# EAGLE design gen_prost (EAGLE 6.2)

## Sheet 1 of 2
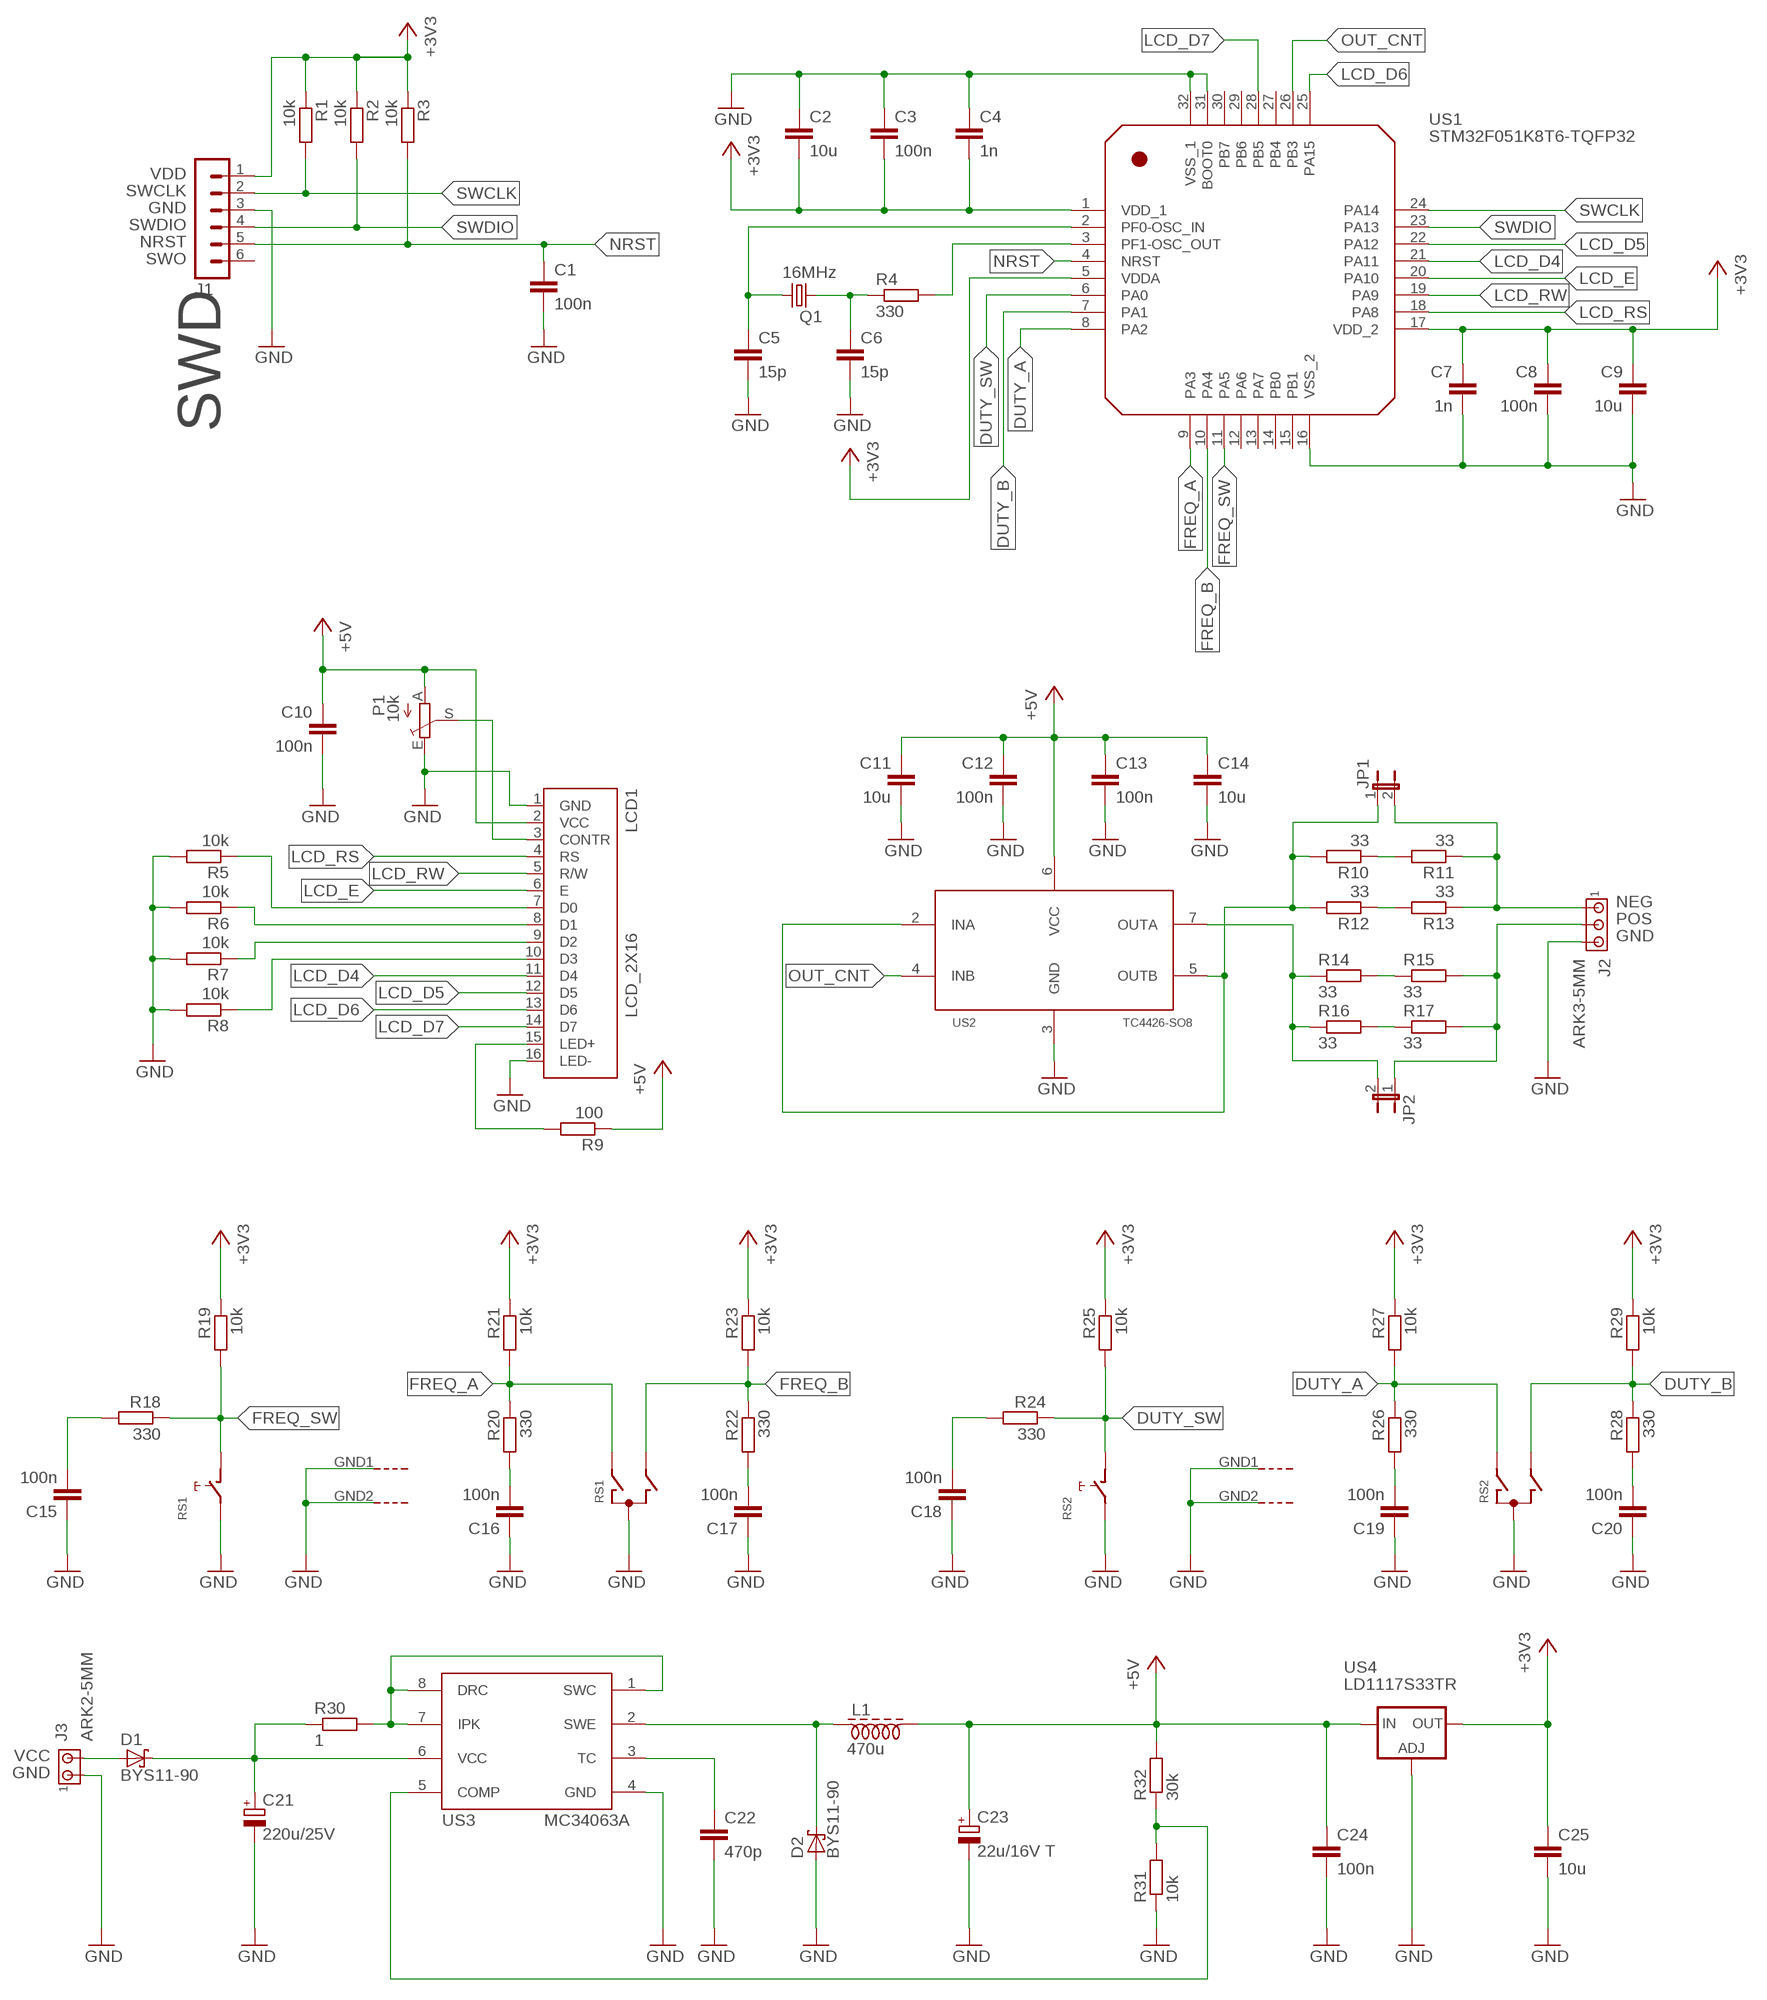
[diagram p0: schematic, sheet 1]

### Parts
C1  100n  C-EUC0805K  [C0805K]
C2  10u  C-EUC0805K  [C0805K]
C3  100n  C-EUC0805K  [C0805K]
C4  1n  C-EUC0805K  [C0805K]
C5  15p  C-EUC0805K  [C0805K]
C6  15p  C-EUC0805K  [C0805K]
C7  1n  C-EUC0805K  [C0805K]
C8  100n  C-EUC0805K  [C0805K]
C9  10u  C-EUC0805K  [C0805K]
C10  100n  C-EUC0805K  [C0805K]
C11  10u  C-EUC0805K  [C0805K]
C12  100n  C-EUC0805K  [C0805K]
C13  100n  C-EUC0805K  [C0805K]
C14  10u  C-EUC0805K  [C0805K]
C15  100n  C-EUC0805K  [C0805K]
C16  100n  C-EUC0805K  [C0805K]
C17  100n  C-EUC0805K  [C0805K]
C18  100n  C-EUC0805K  [C0805K]
C19  100n  C-EUC0805K  [C0805K]
C20  100n  C-EUC0805K  [C0805K]
C21  220u/25V  CPOL-EUTT5D7L  [TT5D7L]
C22  470p  C-EUC0805  [C0805]
C23  22u/16V T  CPOL-EUSMCC  [SMC_C]
C24  100n  C-EUC0805K  [C0805K]
C25  10u  C-EUC0805K  [C0805K]
D1  BYS11-90  SCHOTTKY-DIODESMD  [SMB]
D2  BYS11-90  SCHOTTKY-DIODESMD  [SMB]
J1  MA06-1  [MA06-1]
J2  ARK3-5MM  [3PIN-5MM]
J3  ARK2-5MM  [2PIN-5MM]
JP1  JP1E  [JP1]
JP2  JP1E  [JP1]
L1  470u  DLAWIK-PION  [L_PION]
LCD1  LCD_2X16  LCD_2X16-NAD-ELEMENTAMI  [LCD_HD44780_2X16_NAD-ELEMENTAMI]
P1  10k  TRIM_EU-CA6V  [CA6V]
Q1  16MHz  CRYSTALSM49  [SM49]
R1  10k  R-EU_M0805  [M0805]
R2  10k  R-EU_M0805  [M0805]
R3  10k  R-EU_M0805  [M0805]
R4  330  R-EU_M0805  [M0805]
R5  10k  R-EU_M0805  [M0805]
R6  10k  R-EU_M0805  [M0805]
R7  10k  R-EU_M0805  [M0805]
R8  10k  R-EU_M0805  [M0805]
R9  100  R-EU_M0805  [M0805]
R10  33  R-EU_M0805  [M0805]
R11  33  R-EU_M0805  [M0805]
R12  33  R-EU_M0805  [M0805]
R13  33  R-EU_M0805  [M0805]
R14  33  R-EU_M0805  [M0805]
R15  33  R-EU_M0805  [M0805]
R16  33  R-EU_M0805  [M0805]
R17  33  R-EU_M0805  [M0805]
R18  330  R-EU_M0805  [M0805]
R19  10k  R-EU_M0805  [M0805]
R20  330  R-EU_M0805  [M0805]
R21  10k  R-EU_M0805  [M0805]
R22  330  R-EU_M0805  [M0805]
R23  10k  R-EU_M0805  [M0805]
R24  330  R-EU_M0805  [M0805]
R25  10k  R-EU_M0805  [M0805]
R26  330  R-EU_M0805  [M0805]
R27  10k  R-EU_M0805  [M0805]
R28  330  R-EU_M0805  [M0805]
R29  10k  R-EU_M0805  [M0805]
R30  1  R-EU_M0805  [M0805]
R31  10k  R-EU_M0805  [M0805]
R32  30k  R-EU_M0805  [M0805]
RS1  EC12E_SW  [ALPS_EC12E_SW]
RS2  EC12E_SW  [ALPS_EC12E_SW]
US1  STM32F051K8T6-TQFP32  STM32F051-TQFP32  [TQFP32]
US2  TC4426-SO8  [SO08]
US3  MC34063A  MC34063-SO8  [SO08@1]
US4  LD1117S33TR  LD117AS33TR  [SOT223]

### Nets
+3V3: C2.2 C3.2 C4.2 C7.1 C8.1 C9.1 C25.1 J1.1 R1.1 R2.1 R3.1 R19.1 R21.1 R23.1 R25.1 R27.1 R29.1 US1.1(VDD_1) US1.5(VDDA) US1.17(VDD_2) US4.4(OUT)
+5V: C10.1 C11.1 C12.1 C13.1 C14.1 C23.+ C24.1 L1.P$2 LCD1.2(VCC) P1.A R9.1 R32.2 US2.6(VCC) US4.3(IN)
DUTY_A: R26.1 R27.2 RS2.A US1.8(PA2)
DUTY_B: R28.1 R29.2 RS2.B US1.7(PA1)
DUTY_SW: R24.1 R25.2 RS2.D US1.6(PA0)
FREQ_A: R20.1 R21.2 RS1.A US1.9(PA3)
FREQ_B: R22.1 R23.2 RS1.B US1.10(PA4)
FREQ_SW: R18.1 R19.2 RS1.D US1.11(PA5)
GND: C1.2 C2.1 C3.1 C4.1 C5.2 C6.2 C7.2 C8.2 C9.2 C10.2 C11.2 C12.2 C13.2 C14.2 C15.1 C16.1 C17.1 C18.1 C19.1 C20.1 C21.- C22.2 C23.- C24.2 C25.2 D2.A J1.3 J2.P$3 J3.P$1 LCD1.1(GND) LCD1.16(LED-) P1.E R5.2 R6.2 R7.2 R8.2 R31.1 RS1.C RS1.E RS1.GND1(G) RS1.GND2(G) RS2.C RS2.E RS2.GND1(G) RS2.GND2(G) US1.16(VSS_2) US1.31(BOOT0) US1.32(VSS_1) US2.3(GND) US3.4(GND) US4.1(ADJ)
LCD_D4: LCD1.11(D4) US1.21(PA11)
LCD_D5: LCD1.12(D5) US1.22(PA12)
LCD_D6: LCD1.13(D6) US1.25(PA15)
LCD_D7: LCD1.14(D7) US1.28(PB5)
LCD_E: LCD1.6(E) US1.20(PA10)
LCD_RS: LCD1.4(RS) US1.18(PA8)
LCD_RW: LCD1.5(R/W) US1.19(PA9)
N$1: R31.2 R32.1 US3.5(COMP)
N$2: C18.2 R24.2
N$3: C19.2 R26.2
N$4: C20.2 R28.2
N$5: JP2.2 R14.1 R16.1 US2.7(OUTA)
N$6: R10.1 R11.2
N$7: R12.1 R13.2
N$8: J2.P$1 JP1.2 R11.1 R13.1
N$9: JP1.1 R10.2 R12.2 US2.2(INA) US2.5(OUTB)
N$10: C15.2 R18.2
N$11: J2.P$2 JP2.1 R15.2 R17.2
N$12: C16.2 R20.2
N$13: C17.2 R22.2
N$14: LCD1.9(D2) R7.1
N$16: R16.2 R17.1
N$17: R14.2 R15.1
N$23: C5.1 Q1.1 US1.2(PF0-OSC_IN)
N$24: LCD1.15(LED+) R9.2
N$25: LCD1.3(CONTR) P1.S
N$26: LCD1.8(D1) R6.1
N$27: LCD1.7(D0) R5.1
N$28: LCD1.10(D3) R8.1
N$31: D1.A J3.P$2
N$32: C21.+ D1.C R30.1 US3.6(VCC)
N$37: R30.2 US3.1(SWC) US3.7(IPK) US3.8(DRC)
N$38: C22.1 US3.3(TC)
N$39: D2.C L1.P$1 US3.2(SWE)
N$71: R4.2 US1.3(PF1-OSC_OUT)
N$72: C6.1 Q1.2 R4.1
NRST: C1.1 J1.5 R3.2 US1.4(NRST)
OUT_CNT: US1.26(PB3) US2.4(INB)
SWCLK: J1.2 R1.2 US1.24(PA14)
SWDIO: J1.4 R2.2 US1.23(PA13)
Unconnected: J1.6 US1.12(PA6) US1.13(PA7) US1.14(PB0) US1.15(PB1) US1.27(PB4) US1.29(PB6) US1.30(PB7)

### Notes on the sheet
- VDD
- SWCLK
- GND
- SWDIO
- NRST
- SWO
- SWD
- NEG
- POS
- GND
- VCC
- GND

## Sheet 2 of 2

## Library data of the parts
C1-C20 C22 C24 C25 = rcl:C-EU: CAPACITOR, European symbol
C21 C23 = rcl:CPOL-EU: POLARIZED CAPACITOR, European symbol
D1 D2 = diode:SCHOTTKY-DIODE: Schottky Diode
J1 = con-lstb:MA06-1: PIN HEADER; OC_FARNELL: unknown; OC_NEWARK: unknown
J2 = zlacza_futrzak:ARK3: ARK 3 Raster 5mm i 3,5mm
J3 = zlacza_futrzak:ARK2: ARK 2
JP1 JP2 = jumper:JP1E: JUMPER
L1 = inne_futrzak:DLAWIK
LCD1 = inne_futrzak:LCD_2X16
P1 = pot:TRIM_EU-: POTENTIOMETER
Q1 = crystal:CRYSTAL: CRYSTAL; OC_FARNELL: unknown; OC_NEWARK: unknown
R1-R32 = rcl:R-EU_: RESISTOR, European symbol
RS1 RS2 = switch-alps:EC12E_SW: ALPS rotary Encoder EC12E series with switch; MPN: EC12E2424407; OC_FARNELL: 1520813; OC_NEWARK: 74M1068
US1 = scalaki_futrzak:STM32F051-TQFP32
US2 = scalaki_futrzak:TC4426
US3 = scalaki_futrzak:MC34063
US4 = v-reg:LD117A?*: Low drop fixed and adjustable positive voltage regulators 1 A Source: http://www.st.com/stonline/products/literature/ds/7194/ld1117axx.pdf

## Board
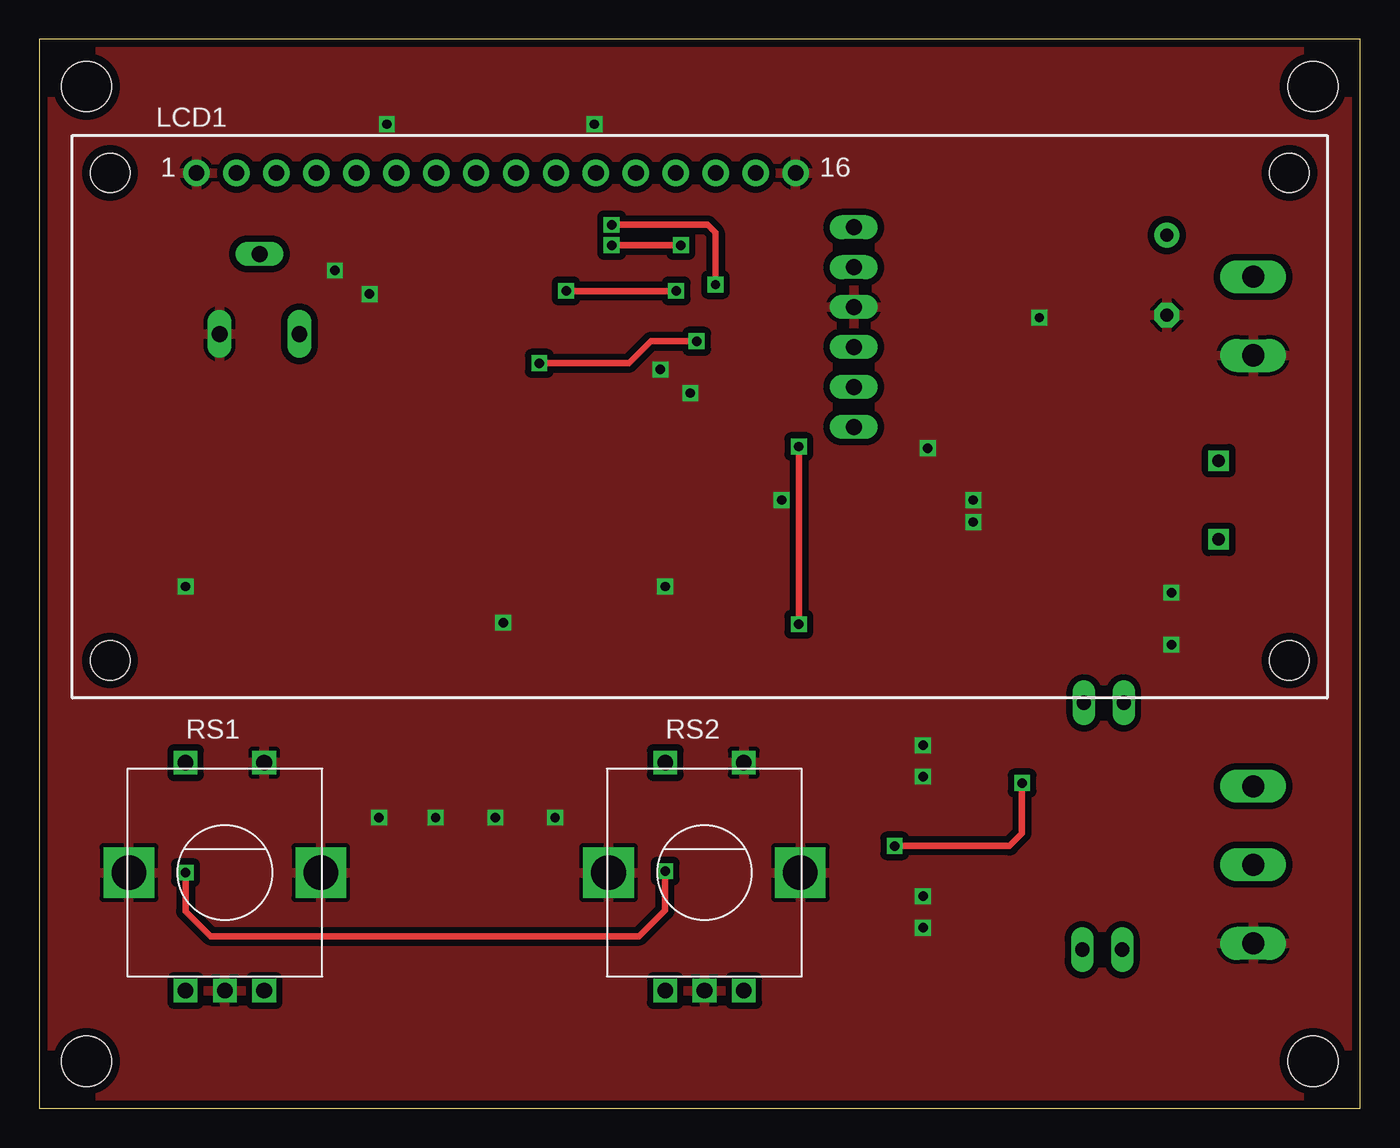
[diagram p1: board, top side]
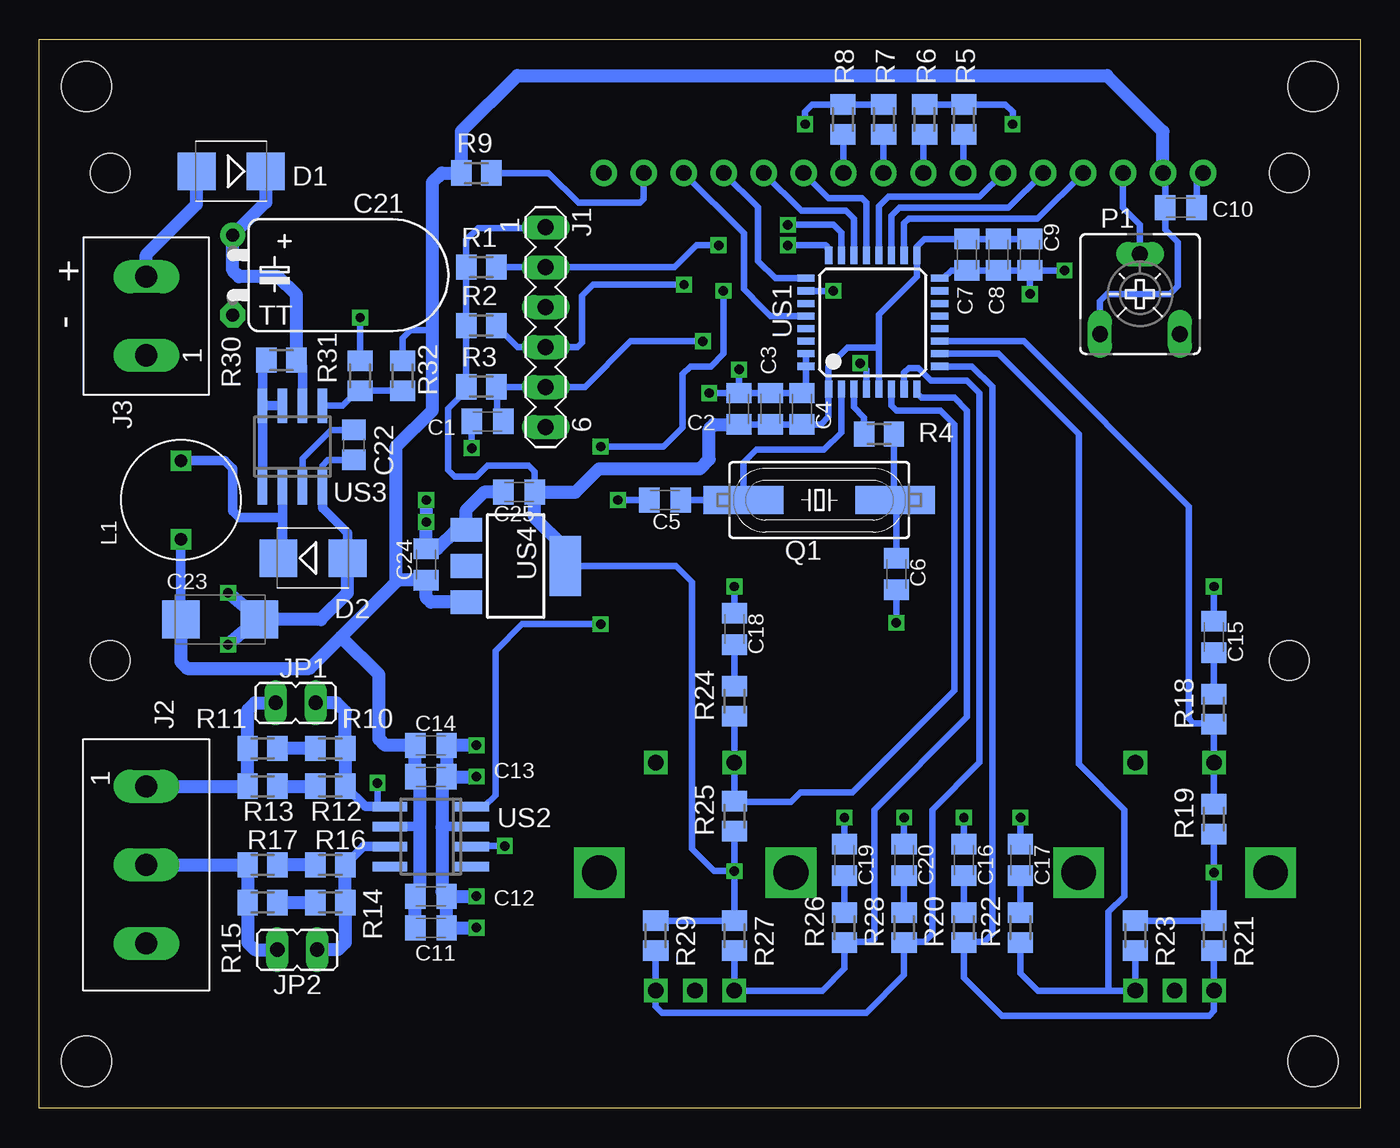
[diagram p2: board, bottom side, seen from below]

Size 84 x 68 mm. Coordinates in mm from the lower left corner, seen from the top.
Outline: 0,0 84,0 84,68 0,68 0,0
Copper layers (1*16): Top 0.035mm / dielectric 1.5mm / Bottom 0.035mm
Design rules: minimum track width 10mil, minimum drill 23mil, track to track 8mil, track to pad 8mil, pad to pad 8mil, via to via 8mil, smd to smd 8mil, copper to edge 20mil, drill to drill 8mil, minimum pad ring 10mil, minimum via ring 8mil, stop-mask expansion 4mil, vias tented up to drill 0mil, thermal gap 10mil
Holes 3.2 mm at 3,3 81,3 3,65 81,65

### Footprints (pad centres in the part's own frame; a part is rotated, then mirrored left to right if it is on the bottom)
C0805K = smd 1.3 x 1.6: 1 -1,0; 2 1,0
TT5D7L = drill 0.813 pad 1.6: + -2.54,0 | drill 0.813 pad 1.6 octagon: - 2.54,0
C0805 = smd 1.3 x 1.5: 1 -0.95,0; 2 0.95,0
SMC_C = smd 2.4 x 2.4: + -2.5,0; - 2.5,0
SMB = smd 2.4 x 2.4: A 2.2,0; C -2.2,0
MA06-1 = drill 1.016 long: 1 -6.35,0; 2 -3.81,0; 3 -1.27,0; 4 1.27,0; 5 3.81,0; 6 6.35,0
3PIN-5MM = drill 1.4 long: P$1 -5,0; P$2 0,0; P$3 5,0
2PIN-5MM = drill 1.4 long: P$1 -2.5,0; P$2 2.5,0
JP1 = drill 0.914 long: 1 0,-1.27; 2 0,1.27
L_PION = drill 0.8 square: P$1 -2.5,0; P$2 2.5,0
LCD_HD44780_2X16_NAD-ELEMENTAMI = drill 1 pad 1.676: 1 -32,15.5; 2 -29.46,15.5; 3 -26.92,15.5; 4 -24.38,15.5; 5 -21.84,15.5; 6 -19.3,15.5; 7 -16.76,15.5; 8 -14.22,15.5; 9 -11.68,15.5; 10 -9.14,15.5; 11 -6.6,15.5; 12 -4.06,15.5; 13 -1.52,15.5; 14 1.02,15.5; 15 3.56,15.5; 16 6.1,15.5 | hole 2.5: -37.5,-15.5; 37.5,-15.5; -37.5,15.5; 37.5,15.5
CA6V = drill 1.016 long: A -2.54,-2.54; E 2.54,-2.54; S 0,2.54
SM49 = smd 5.08 x 1.778: 1 -4.826,0; 2 4.826,0
M0805 = smd 1.3 x 1.6: 1 -0.95,0; 2 0.95,0
ALPS_EC12E_SW = drill 1 square: A -2.5,-7.5; B 2.5,-7.5; C 0,-7.5; D -2.5,7; E 2.5,7 | drill 2.2 square: GND1 -6.1,0; GND2 6.1,0
TQFP32 = smd 1.1 x 0.45: 1 -4.25,2.8; 2 -4.25,2; 3 -4.25,1.2; 4 -4.25,0.4; 5 -4.25,-0.4; 6 -4.25,-1.2; 7 -4.25,-2; 8 -4.25,-2.8; 17 4.25,-2.8; 18 4.25,-2; 19 4.25,-1.2; 20 4.25,-0.4; 21 4.25,0.4; 22 4.25,1.2; 23 4.25,2; 24 4.25,2.8 | smd 0.45 x 1.1: 9 -2.8,-4.25; 10 -2,-4.25; 11 -1.2,-4.25; 12 -0.4,-4.25; 13 0.4,-4.25; 14 1.2,-4.25; 15 2,-4.25; 16 2.8,-4.25; 25 2.8,4.25; 26 2,4.25; 27 1.2,4.25; 28 0.4,4.25; 29 -0.4,4.25; 30 -1.2,4.25; 31 -2,4.25; 32 -2.8,4.25
SO08 = smd 0.6 x 2.2: 1 -1.905,-2.6; 2 -0.635,-2.6; 3 0.635,-2.6; 4 1.905,-2.6; 5 1.905,2.6; 6 0.635,2.6; 7 -0.635,2.6; 8 -1.905,2.6
SO08@1 = smd 0.6 x 2.2: 1 -1.905,-2.6; 2 -0.635,-2.6; 3 0.635,-2.6; 4 1.905,-2.6; 5 1.905,2.6; 6 0.635,2.6; 7 -0.635,2.6; 8 -1.905,2.6
SOT223 = smd 1.5 x 2: 1 -2.3,-3.15; 2 0,-3.15; 3 2.3,-3.15 | smd 3.8 x 2: 4 0,3.15

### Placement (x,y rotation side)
C1  55.5,43.7 180 bottom
C2  39.5,44.5 270 bottom
C3  37.5,44.5 270 bottom
C4  35.5,44.5 270 bottom
C5  44.2,38.7 180 bottom
C6  29.5,34 270 bottom
C7  25,54.3 270 bottom
C8  23,54.3 270 bottom
C9  21,54.3 270 bottom
C10  11.4,57.3 0 bottom
C11  59.1,11.5 0 bottom
C12  59.1,13.5 0 bottom
C13  59.1,21.1 0 bottom
C14  59.1,23.1 0 bottom
C15  9.3,30 270 bottom
C16  25.2,15.8 270 bottom
C17  21.6,15.8 270 bottom
C18  39.8,30.5 270 bottom
C19  32.8,15.8 270 bottom
C20  29,15.8 270 bottom
C21  71.7,53 270 bottom
C22  64,42.2 270 bottom
C23  72.5,31.1 0 bottom
C24  59.4,34.6 90 bottom
C25  53.5,39.2 180 bottom
D1  71.8,59.6 180 bottom
D2  66.6,35 0 bottom
J1  51.8,49.7 270 bottom
J2  77.2,15.5 270 bottom
J3  77.2,50.4 90 bottom
JP1  67.7,25.8 90 bottom
JP2  67.6,10.1 270 bottom
L1  75,38.7 270 bottom
LCD1  42,44 0 top
P1  14,51.8 0 bottom
Q1  34.4,38.7 0 bottom
R1  55.9,53.5 0 bottom
R2  55.9,49.8 0 bottom
R3  55.9,45.9 0 bottom
R4  30.6,42.9 180 bottom
R5  25.2,62.9 90 bottom
R6  27.7,62.9 90 bottom
R7  30.3,62.9 90 bottom
R8  32.9,62.9 90 bottom
R9  56.2,59.5 0 bottom
R10  65.5,22.9 0 bottom
R11  69.8,22.9 0 bottom
R12  65.5,20.5 0 bottom
R13  69.8,20.5 0 bottom
R14  65.5,13.1 180 bottom
R15  69.8,13.1 180 bottom
R16  65.5,15.5 180 bottom
R17  69.8,15.5 180 bottom
R18  9.3,25.4 90 bottom
R19  9.3,18.4 90 bottom
R20  25.2,11.5 90 bottom
R21  9.3,11 270 bottom
R22  21.6,11.5 90 bottom
R23  14.3,11 270 bottom
R24  39.8,25.9 90 bottom
R25  39.8,18.6 90 bottom
R26  32.8,11.5 90 bottom
R27  39.8,11 270 bottom
R28  29,11.5 90 bottom
R29  44.8,11 270 bottom
R30  68.6,47.6 180 bottom
R31  63.6,46.6 270 bottom
R32  60.9,46.6 90 bottom
RS1  11.8,15 0 top
RS2  42.3,15 0 top
US1  31,50 90 bottom
US2  59.1,17.3 90 bottom
US3  67.9,42.1 0 bottom
US4  53.7,34.5 270 bottom

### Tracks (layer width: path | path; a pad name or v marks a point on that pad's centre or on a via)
+3V3  (via drill 0.6)
  Top 0.406: v9.3,15 9.3,12.55 10.9,10.95 38.15,10.95 39.8,12.6 v39.8,15.1
  Bottom 0.406: C2.2 C3.2 C4.2 34.3,43.5 33.8,44 US1.1 33.8,47.2 32.6,48.4 30.6,48.4 | 30.6,48.4 30.6,50.5 28.2,52.9 US1.17 28.2,54.8 27.7,55.3 C7.1 C8.1 C9.1 | 30.6,48.4 US1.5 | J1.1 51.85,56 56.1,56 56.85,55.25 R1.1 R2.1 R3.1 57.2,45.55 57.2,45.3 58,44.5 58,40.6 57.6,40.2 56.2,40.2 55.5,40.9 52.9,40.9 52.5,40.5 C25.1 | R23.1 R21.1 v9.3,15 R19.1 | v39.8,15.1 R25.1 | R29.1 R27.1 v39.8,15.1 | US4.4 43.5,34.5 42.5,33.5 42.5,16.5 41.1,15.1 v39.8,15.1
  Bottom 0.813: US4.4 50.55,35.65 52.5,37.6 C25.1 49.9,39.2 48.4,40.7 42,40.7 41.4,41.3 41.4,43.2 41.1,43.5 C2.2
+5V
  Bottom 0.406: LCD1.2 12.4,59.36 C10.1 12.4,55.9 11.6,55.1 11.6,52.3 12.1,51.8 16.1,51.8 16.54,51.36 P1.A | R32.2 60.9,49 60.4,49.5 59,49.5
  Bottom 0.61: L1.P$2 C23.+ | US2.6 59.84,17.93 59.8,17.9
  Bottom 0.813: C23.+ 75,28.4 74.6,28 66.8,28 64.8,30 | 64.8,30 61.3,33.5 | 61.3,33.5 61.3,42.1 59,44.4 59,49.5 59,58.9 58.4,59.5 R9.1 57.15,62.15 53.6,65.7 16.1,65.7 12.54,62.14 LCD1.2 | US4.3 59.1,32.2 59.4,32.5 C24.1 61.2,33.6 61.3,33.5 | 64.8,30 62.4,27.6 62.4,23.5 62,23.1 C14.1 C13.1 59.8,20.8 59.8,17.9 59.8,14.1 60.1,13.8 C12.1 C11.1
DUTY_A
  Bottom 0.406: R27.2 RS2.A 34.2,7.5 32.8,8.9 R26.1 32.75,10.6 31.1,10.6 30.9,10.8 30.9,19 25,24.9 25,44.4 25.8,45.2 27.9,45.2 28.2,45.5 US1.8
DUTY_B
  Bottom 0.406: R29.2 RS2.B 44.8,6.5 44.4,6.1 31.4,6.1 29,8.5 R28.1 28.95,10.6 27.7,10.6 27.2,11.1 27.2,19 24.2,22 24.2,45.5 25,46.3 27.3,46.3 28.1,47.1 28.7,47.1 29,46.8 US1.7
DUTY_SW
  Bottom 0.406: R24.1 RS2.D R25.2 39.75,19.5 36.2,19.5 35.6,20.1 32.3,20.1 25.8,26.6 25.8,43.5 26.7,44.4 29.5,44.4 29.8,44.7 US1.6
FREQ_A
  Bottom 0.406: R21.2 RS1.A 9.3,6.2 9.6,5.9 22.8,5.9 25.2,8.3 R20.1 25.15,10.6 23.9,10.6 23.4,11.1 23.4,45.9 24.7,47.2 US1.9
FREQ_B
  Bottom 0.406: 16,7.5 RS1.B R23.2 14.25,10 | 16,7.5 20.5,7.5 21.6,8.6 R22.1 | US1.10 23,48 17.9,42.9 17.9,21.9 15,19 15,13.5 16,12.5 16,7.5
FREQ_SW
  Bottom 0.406: R19.2 RS1.D R18.1 9.35,24.5 10.6,24.5 10.9,24.8 10.9,38.3 21.4,48.8 US1.11
GND  (via drill 0.6)
  Bottom 0.406: C2.1 C3.1 C4.1 35.25,45.75 US1.32 US1.31 | C2.1 v39.5,47 | v41.4,45.5 C2.1 | C5.2 v47.2,38.7 | US1.16 26.5,52.8 26,53.3 C7.2 C8.2 C9.2 | C9.2 v21,51.8 | v18.8,53.3 C9.2 | v22.1,62.6 22.1,63.4 22.55,63.85 R5.2 R6.2 | v35.3,62.6 35.3,63.4 34.85,63.85 R8.2 R7.2 | C10.2 10.4,59.1 LCD1.1 | C1.2 v56.5,42 | US3.4 66,40.91 65.65,41.25 C22.2 | R31.1 v63.6,50.3 | C17.1 v21.6,18.5 | v32.8,18.5 C19.1 | C20.1 v29,18.5 | C16.1 v25.2,18.5 | C18.1 v39.8,33.2 | v9.3,33.2 C15.1 | v29.5,30.9 C6.2
  Bottom 0.61: US3.4 66,38.2 64.4,36.6 D2.A | US2.3 58.37,17.93 58.4,17.9
  Bottom 0.813: D2.A 64.4,32.8 66.1,31.1 C23.- | C23.- v72,32.8 | C23.- 70.1,31.1 v72,29.5 | v59.4,38.7 v59.4,37.3 C24.2 58.7,35.6 57.5,36.8 US4.1 56.85,38.05 55.7,39.2 C25.2 | v56.2,11.5 C11.2 C12.2 | C12.2 v56.2,13.5 | C13.2 58.1,20.8 58.4,20.5 58.4,17.9 58.4,13.8 C12.2 | C13.2 v56.2,21.1 | v56.2,23.1 C14.2 C13.2
  pour Top (isolate 0.406): 0,0 84,0 84,68 0,68
LCD_D4
  Bottom 0.406: US1.21 31.4,57.6 31.7,57.9 33.8,57.9 LCD1.11
LCD_D5
  Bottom 0.406: US1.22 32.2,56.6 32.7,57.1 35.54,57.1 LCD1.12
LCD_D6
  Bottom 0.406: US1.25 37.2,52.8 38.3,53.9 38.3,57.32 LCD1.13
LCD_D7
  Bottom 0.406: LCD1.14 39.2,55.68 39.2,52.1 38.05,50.95 37.6,50.5 37.5,50.4 US1.28
LCD_E
  Bottom 0.406: US1.20 30.6,57.4 30,58 24.2,58 LCD1.6
LCD_RS
  Bottom 0.406: US1.18 29,56.3 28.7,56.6 20.52,56.6 LCD1.4
LCD_RW
  Bottom 0.406: US1.19 29.8,56.8 29.3,57.3 22.36,57.3 LCD1.5
N$1
  Bottom 0.406: R32.1 R31.2 63.75,45.65 64.7,44.7 US3.5
N$2
  Bottom 0.406: C18.2 R24.2
N$3
  Bottom 0.406: R26.2 C19.2
N$4
  Bottom 0.406: R28.2 C20.2
N$5
  Bottom 0.61: US2.7 63.38,16.66 R16.1
  Bottom 0.813: JP2.2 65,10.1 64.55,10.55 R14.1 R16.1
N$6
  Bottom 0.813: R10.1 R11.2
N$7
  Bottom 0.813: R13.2 R12.1
N$8
  Bottom 0.813: J2.P$1 R13.1 R11.1 70.75,25.35 70.3,25.8 JP1.2
N$9  (via drill 0.6)
  Top 0.406: v62.5,20.7 62.5,17.5 61.7,16.7 v54.4,16.7
  Bottom 0.406: US2.5 62.49,19.2 62.5,19.2 v62.5,20.7 | v54.4,16.7 56.47,16.7 US2.2
  Bottom 0.61: US2.5 63.26,19.2 R12.2
  Bottom 0.813: JP1.1 65.1,25.8 64.55,25.25 R10.2 R12.2
N$10
  Bottom 0.406: C15.2 R18.2
N$11
  Bottom 0.813: J2.P$2 R17.2 R15.2 70.75,10.55 70.3,10.1 JP2.1
N$12
  Bottom 0.406: R20.2 C16.2
N$13
  Bottom 0.406: R22.2 C17.2
N$14
  Bottom 0.406: LCD1.9 30.32,61.93 R7.1
N$16
  Bottom 0.813: R16.2 R17.1
N$17
  Bottom 0.813: R15.1 R14.2
N$23
  Bottom 0.406: US1.2 33,43 34.1,41.9 38.4,41.9 39.23,41.07 Q1.1 C5.1
N$24
  Bottom 0.406: LCD1.15 45.56,57.84 45.8,57.6 49.7,57.6 51.6,59.5 R9.2
N$25
  Bottom 0.406: LCD1.3 15.08,57.28 14,56.2 P1.S
N$26
  Bottom 0.406: LCD1.8 27.78,61.87 R6.1
N$27
  Bottom 0.406: LCD1.7 25.24,61.91 R5.1
N$28
  Bottom 0.406: LCD1.10 32.86,61.91 R8.1
N$31
  Bottom 0.813: J3.P$2 77.2,54.3 74,57.5 D1.A
N$32
  Bottom 0.61: US3.6 67.27,47.22 R30.1
  Bottom 0.813: D1.C 69.6,57.64 C21.+ 71.7,53.3 71.3,52.9 68.8,52.9 67.65,51.75 R30.1
N$37
  Bottom 0.61: US3.8 69.81,47.34 R30.2 | US3.7 US3.8 | US3.1 US3.8
N$38
  Bottom 0.406: C22.1 65.45,43.15 67.27,41.34 US3.3
N$39
  Bottom 0.61: US3.2 68.53,37.6 | 68.53,37.6 68.53,35.27 D2.C | L1.P$1 72.2,41.2 71.7,40.7 71.7,38 71.3,37.6 68.53,37.6
N$71
  Bottom 0.406: US1.3 32.2,44.6 31.55,43.95 R4.2
N$72
  Bottom 0.406: R4.1 29.65,38.78 Q1.2 29.5,38.63 C6.1
NRST  (via drill 0.6)
  Top 0.406: v31.8,47.4 37.5,47.4 38.9,48.8 v41.8,48.8
  Bottom 0.406: US1.4 31.4,47 v31.8,47.4 | v41.8,48.8 46.4,48.8 49.31,45.89 J1.5 R3.2 54.9,45.85 54.9,44.1 C1.1
OUT_CNT  (via drill 0.6)
  Top 0.406: v48.3,42.1 v48.3,30.8 | v40.5,52 v33.5,52
  Bottom 0.406: v48.3,42.1 44.3,42.1 43.1,43.3 43.1,46.7 42.6,47.2 41.3,47.2 40.5,48 v40.5,52 | v48.3,30.8 53.3,30.8 55,29.1 55,19.9 55.7,19.2 US2.4 | v33.5,52 US1.26
SWCLK  (via drill 0.6)
  Top 0.406: v36.4,54.9 v40.8,54.9
  Bottom 0.406: R1.2 J1.2 43.6,53.5 42.2,54.9 v40.8,54.9 | US1.24 33.8,54.7 34,54.9 v36.4,54.9
SWDIO  (via drill 0.6)
  Top 0.406: v36.4,56.2 42.5,56.2 43,55.7 v43,52.4
  Bottom 0.406: R2.2 53.58,48.43 J1.4 49.77,48.43 49.5,48.7 49.5,51.7 48.8,52.4 v43,52.4 | US1.23 33,55.7 33.5,56.2 v36.4,56.2

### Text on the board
bPlace: + -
